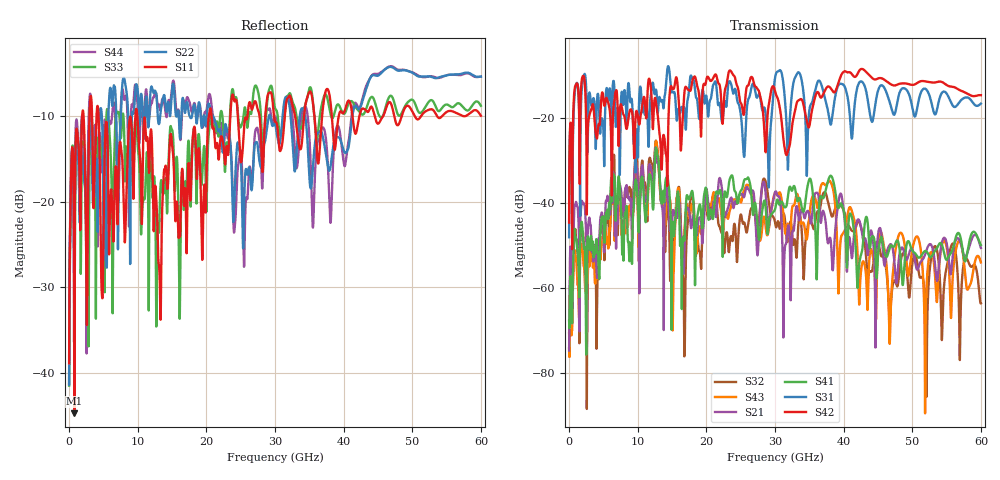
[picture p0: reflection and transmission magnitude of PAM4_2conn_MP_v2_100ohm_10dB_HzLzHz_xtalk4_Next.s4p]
! Info: Touchstone file created by Circ.  Input file=FAB50GbE_2conn_Midplane_Examax_Topo2_v2_100ohm_10dB_HzLzHz.circ
# Hz S RI R 50
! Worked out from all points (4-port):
!   6000 points, 10 MHz to 60 GHz, reference 50 ohm
!   strongest paths, dB at 10 MHz, 15.01 GHz, 30.01 GHz, 45.01 GHz, 60 GHz:
!     S42: -44.6, -12.9, -13.6, -10.6, -14.5
!     S31: -48.1, -13.8, -10.5, -13.5, -16.5
!     S41: -67.8, -47.8, -41.4, -52.4, -49.9
!     S21: -74.8, -45.1, -37.4, -47.6, -50.6
!     S43: -70.8, -54.3, -37.5, -51.2, -54.0
!     S32: -74.3, -54.4, -44.5, -49.3, -63.7
!   lowest |S11| = -44.6 dB at 770 MHz (marker M1), VSWR 1.01, Z = 50 - j0.586 ohm
!   |S11| at or under -10 dB: 4.294 GHz to 9.665 GHz (5.372 GHz wide, 77 % of centre); 9.942 GHz to 20.38 GHz (10.44 GHz wide, 68.8 % of centre); 20.75 GHz to 23.49 GHz (2.734 GHz wide, 12.4 % of centre)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
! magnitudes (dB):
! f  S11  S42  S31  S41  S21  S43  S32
! 10 MHz  -38.8  -44.6  -48.1  -67.8  -74.8  -70.8  -74.3
! 770 MHz  -44.6  -13.7  -15.2  -46.4  -41.0  -51.5  -48.0
! 12.74 GHz  -20.1  -17.2  -13.8  -27.2  -28.4  -25.7  -25.9
! 16.77 GHz  -20.3  -14.6  -17.4  -48.7  -53.5  -46.9  -70.9
! 17.81 GHz  -16.8  -12.7  -10.0  -37.6  -45.9  -40.8  -38.8
! 28.45 GHz  -12.1  -22.9  -17.5  -39.4  -35.3  -43.3  -34.3
! 60 GHz  -10.0  -14.5  -16.5  -49.9  -50.6  -54.0  -63.7
